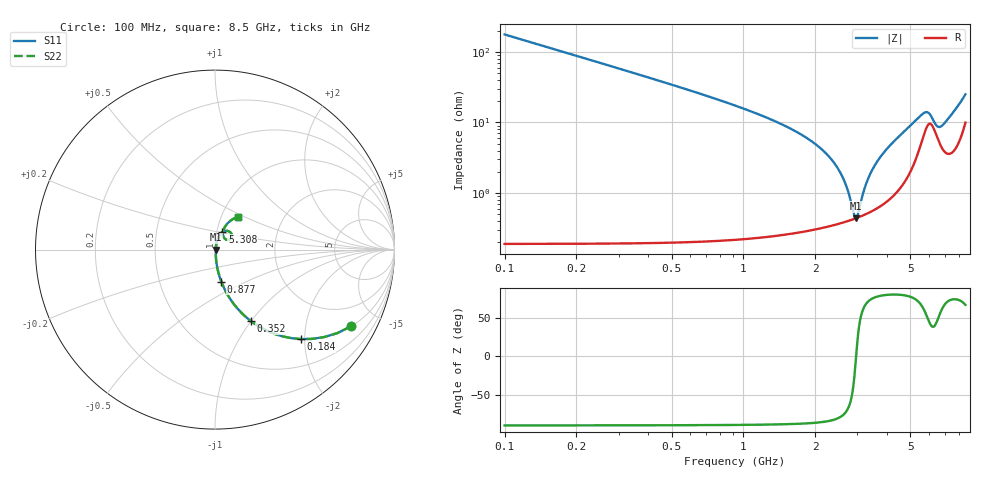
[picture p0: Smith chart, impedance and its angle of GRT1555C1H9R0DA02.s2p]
!Murata Part Number: GRT1555C1H9R0DA02
!These Parameters are Measured in Series Mode Connection
!Data Generated on Jun 19, 2026
!  o--ll--o
!Port1  Port2
!  o------o
!Operation Temp=25[degC], DC Bias Voltage=0[V]
!Freq. Start=100[MHz] Stop=9[GHz] 401[Steps]
# Hz S RI R 50
!Freq.(Hz) S11(Real) S11(Imag) S21(Real) S21(Imag) S12(Real) S12(Imag) S22(Real) S22(Imag)
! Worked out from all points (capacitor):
!   401 points, 100 MHz to 8.5 GHz, reference 50 ohm
!   read as one part in series: C = 9 pF near 142 MHz
!   lowest |Z| = 441 mohm at 2.956 GHz (marker M1)
!   series resonance near 2.964 GHz, so ESL is about 320 pH
!   S11 on the Smith chart (normalised r, x): 100 MHz: 1.00, -3.53; 184 MHz: 1.00, -1.92; 352 MHz: 1.00, -0.99; 877 MHz: 1.00, -0.37; 5.308 GHz: 1.06, +0.21; 8.5 GHz: 1.20, +0.46
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1e8  0.7571 -0.4283  0.2429 0.4283  0.2429 0.4283  0.7571 -0.4283
1.84e8  0.4784 -0.4985  0.5216 0.4985  0.5216 0.4985  0.4784 -0.4985
3.52e8  0.1982 -0.3967  0.8018 0.3967  0.8018 0.3967  0.1982 -0.3967
5.41e8  0.0925 -0.2866  0.9075 0.2866  0.9075 0.2866  0.0925 -0.2866
8.77e8  0.035 -0.178  0.965 0.178  0.965 0.178  0.035 -0.178
1.507e9  0.0102 -0.0871  0.9898 0.0871  0.9898 0.0871  0.0102 -0.0871
2.074e9  0.0051 -0.0444  0.9949 0.0444  0.9949 0.0444  0.0051 -0.0444
2.431e9  0.00416 -0.0246  0.9958 0.0246  0.9958 0.0246  0.00416 -0.0246
2.683e9  0.00407 -0.0125  0.9959 0.0125  0.9959 0.0125  0.00407 -0.0125
2.914e9  0.0043 -0.00215  0.9957 0.00215  0.9957 0.00215  0.0043 -0.00215
2.956e9  0.00437 -0.000345  0.9956 0.000345  0.9956 0.000345  0.00437 -0.000345
3.019e9  0.0045 0.00233  0.9955 -0.00233  0.9955 -0.00233  0.0045 0.00233
3.25e9  0.00513 0.0119  0.9949 -0.0119  0.9949 -0.0119  0.00513 0.0119
3.46e9  0.00594 0.0202  0.9941 -0.0202  0.9941 -0.0202  0.00594 0.0202
3.817e9  0.00793 0.0342  0.9921 -0.0342  0.9921 -0.0342  0.00793 0.0342
4.3e9  0.0123 0.0534  0.9877 -0.0534  0.9877 -0.0534  0.0123 0.0534
5.308e9  0.0412 0.0977  0.9588 -0.0977  0.9588 -0.0977  0.0412 0.0977
5.707e9  0.0752 0.1027  0.9248 -0.1027  0.9248 -0.1027  0.0752 0.1027
5.98e9  0.0939 0.0797  0.9061 -0.0797  0.9061 -0.0797  0.0939 0.0797
6.526e9  0.058 0.0582  0.942 -0.0582  0.942 -0.0582  0.058 0.0582
7.114e9  0.0442 0.0934  0.9558 -0.0934  0.9558 -0.0934  0.0442 0.0934
8.5e9  0.1287 0.1826  0.8713 -0.1826  0.8713 -0.1826  0.1287 0.1826
